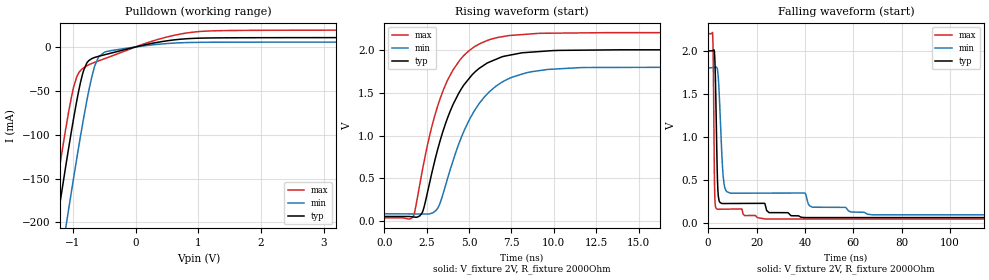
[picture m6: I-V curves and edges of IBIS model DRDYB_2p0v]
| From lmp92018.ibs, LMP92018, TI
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|   Model
[Model]   DRDYB_2p0v
Model_type   Open_drain
Polarity   Non-Inverting
Vmeas = 1
Vref = 1
Cref = 1pF
Rref = 2000
|   typ   min   max
C_comp   0.6389pF   0.6288pF   0.7669pF
[Voltage Range]   2   1.8   2.2
[Temperature Range]   27   125   -40
[Pullup Reference]   2   1.8   2.2
[Pulldown Reference]   0   0   0
[Power Clamp Reference]   2   1.8   2.2
[GND Clamp Reference]   0   0   0
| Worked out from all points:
|   slope of the pulldown table from 0 to 0.3 V, typ, clamps not added: 65 ohm
|   falling waveform, V_fixture 2V, R_fixture 2000Ohm: 20-80 % time 872ps typ, 2.07ns min, 463ps max; typ from 2 V to 0.057 V
|   rising waveform, V_fixture 2V, R_fixture 2000Ohm: 20-80 % time 2.12ns typ, 2.32ns min, 1.94ns max; typ from 0.057 V to 2 V
[Pulldown]
|   Voltage   I(typ)   I(min)   I(max)
-2V       -557.6mA   -628.2mA   -513.3mA
-1.298V   -219.8mA   -291mA     -175.2mA
-1.25V    -197.4mA   -268.5mA   -153mA
-1.118V   -136.9mA   -207.3mA   -94.16mA
-1.07V    -115.6mA   -185.3mA   -74.33mA
-986mV    -79.84mA   -147.6mA   -44.78mA
-926mV    -56.33mA   -121.3mA   -31.86mA
-830mV    -26.82mA   -81.1mA    -23.75mA
-650mV    -11.91mA   -21.11mA   -17.46mA
-494mV    -8.888mA   -5.837mA   -13.35mA
934mV     9.782mA    5.145mA    16.98mA
3.994V    10.67mA    5.542mA    19.17mA
[Ramp]
R_load = 2000
|   typ   min   max
dV/dt_r   1.1657/2.11e-09   1.02676/2.31731e-09   1.29579/1.938e-09
dV/dt_f   1.1657/8.71954e-10   1.02676/2.06693e-09   1.2958/4.631e-10
[Falling Waveform]
V_fixture = 2V
V_fixture_min = 1.8V
V_fixture_max = 2.2V
R_fixture = 2000Ohm
C_fixture = 0F
|   Time   V(typ)   V(min)   V(max)
0s        2V         1.8V       2.2V
1.911ns   2.001V     1.805V     2.186V
2.167ns   2.006V     1.806V     1.804V
2.726ns   1.93V      1.807V     349.9mV
3.777ns   601.4mV    1.795V     155.8mV
4.565ns   252.3mV    1.516V     154.9mV
6.189ns   221.1mV    552.4mV    155.5mV
9.045ns   221.5mV    343.8mV    156.5mV
67.93ns   57.36mV    89.41mV    40.47mV
300ns     57.17mV    88.73mV    40.34mV
[Rising Waveform]
V_fixture = 2V
V_fixture_min = 1.8V
V_fixture_max = 2.2V
R_fixture = 2000Ohm
C_fixture = 0F
|   Time   V(typ)   V(min)   V(max)
0s        57.17mV    88.73mV    40.34mV
1.603ns   53.83mV    86.69mV    34.55mV
1.769ns   50.41mV    86.48mV    87.01mV
2.23ns    97.5mV     85.9mV     576.7mV
3.154ns   840.7mV    153.5mV    1.346V
4.464ns   1.516V     936.4mV    1.88V
5.336ns   1.737V     1.295V     2.036V
6.189ns   1.854V     1.508V     2.114V
9.043ns   1.976V     1.753V     2.189V
300ns     2V         1.8V       2.2V
